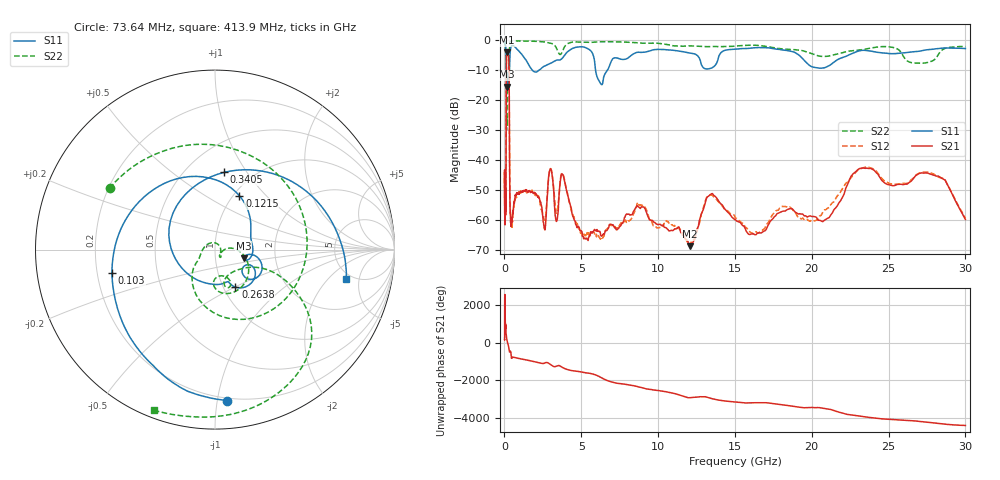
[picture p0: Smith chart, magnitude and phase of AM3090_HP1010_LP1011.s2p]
! Date/Time: Thu, Feb 28, 2019 2:04 PM
! Network Analyzer: Agilent Technologies E8364B Rev: A.07.50.67
! Sweep from 0.010 to 30.000 GHz, 1601 Points, Sweep Type: LOG
! Power Supply: 5.023 V, 0.002 A
# Hz S DB R 50
!freq MagS11 AngS11 MagS21 AngS21 MagS12 AngS12 MagS22 AngS22
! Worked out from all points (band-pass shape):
!   1601 points, 10 MHz to 30 GHz, reference 50 ohm
!   highest |S21| = -4.10 dB at 175 MHz (marker M1); lowest = -68.6 dB at 12.07 GHz (marker M2)
!   |S21| within 3 dB of the highest: 128.2 MHz to 288.1 MHz (159.8 MHz wide, 76.8 % of centre)
!   lowest |S11| = -15.5 dB at 156.8 MHz (marker M3), VSWR 1.40, Z = 68.8 - j6.51 ohm
!   |S11| at or under -10 dB: 122.1 MHz to 326.2 MHz (204.1 MHz wide, 91.1 % of centre); 1.812 GHz to 2.242 GHz (429.8 MHz wide, 21.2 % of centre); 5.927 GHz to 6.709 GHz (781.6 MHz wide, 12.4 % of centre)
!   |S22| runs from -30.0 to -0.2 dB; largest |S21 - S12| = 0.012
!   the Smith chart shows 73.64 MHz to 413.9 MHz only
!   S11 on the Smith chart (normalised r, x): 73.64 MHz: 0.18, -1.07; 103 MHz: 0.26, -0.10; 121.5 MHz: 1.07, +0.72; 263.8 MHz: 1.14, -0.50; 340.5 MHz: 0.75, +0.79; 413.9 MHz: 4.45, -3.30
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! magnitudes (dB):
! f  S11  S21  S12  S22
! 10 MHz  -0.2  -44.1  -47.7  -0.7
! 38.04 MHz  -0.5  -60.3  -60.0  -1.6
! 73.64 MHz  -1.5  -55.0  -51.1  -3.4
! 90.86 MHz  -3.0  -56.7  -51.9  -4.9
! 103 MHz  -4.6  -36.7  -36.5  -5.7
! 121.5 MHz  -9.6  -11.0  -11.0  -12.8
! 144.7 MHz  -13.9  -4.8  -4.8  -27.7
! 156.8 MHz  -15.5  -4.3  -4.3  -23.6
! 175 MHz  -12.3  -4.1  -4.1  -13.6
! 263.8 MHz  -12.5  -5.2  -5.2  -13.3
! 302 MHz  -14.2  -10.8  -10.8  -9.5
! 340.5 MHz  -7.3  -46.1  -45.7  -1.3
! 413.9 MHz  -2.5  -61.4  -59.1  -0.4
! 550.5 MHz  -1.9  -57.8  -57.5  -0.3
! 2.084 GHz  -10.7  -51.4  -52.0  -0.4
! 3.002 GHz  -7.7  -42.9  -42.8  -1.1
! 7.926 GHz  -6.3  -58.0  -60.6  -0.7
! 12.07 GHz  -4.3  -68.6  -68.4  -2.0
! 13.54 GHz  -9.2  -51.1  -51.7  -2.2
! 20.72 GHz  -9.3  -60.4  -57.4  -5.5
! 23.48 GHz  -3.4  -42.7  -42.3  -3.0
! 30 GHz  -2.8  -59.7  -59.3  -2.2
